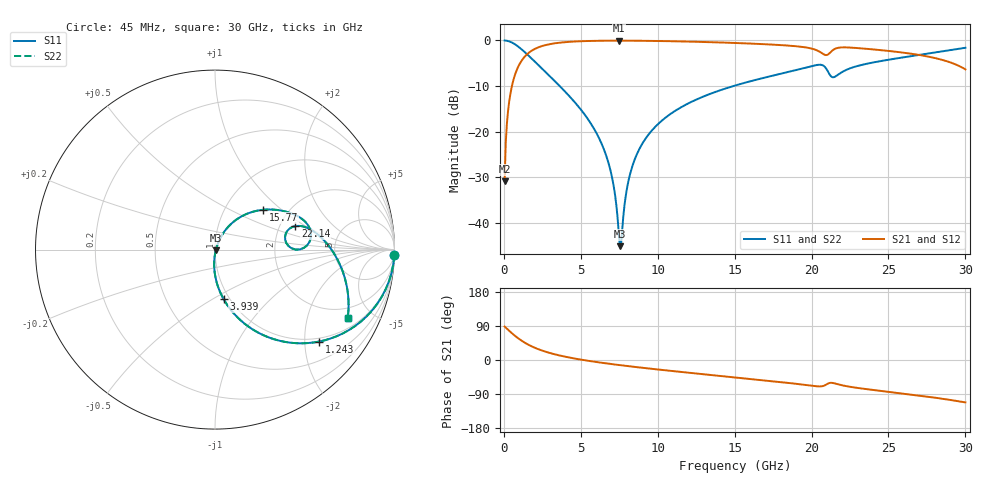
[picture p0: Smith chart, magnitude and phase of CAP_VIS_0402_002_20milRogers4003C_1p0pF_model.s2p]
! S-parameter model data by Modelithics Inc.  support@modelithics.com  813-866-6335  Tampa FL USA
! S-Parameter data specifications:
! Substrate: 20-mil Rogers 4003C, substrate thickness, H=0.508mm, Dielectric constant, Er=3.75
! PCB Mounting Pad Footprint: Pad width, PadW=0.50mm , Pad length, PadL=0.50mm , Pad gap, PadG (edge-to-edge)=0.40mm , Reference planes=1.4mm apart
! Created Wed Nov 18 12:37:36 2015
# hz S ma R 50
! 2 Port Network Data from SP1.SP block
! freq  magS11  angS11  magS21  angS21  magS12  angS12  magS22  angS22
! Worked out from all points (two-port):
!   401 points, 45 MHz to 30 GHz, reference 50 ohm
!   highest |S21| = -0.05 dB at 7.459 GHz (marker M1); lowest = -30.8 dB at 45 MHz (marker M2)
!   |S21| within 3 dB of the highest: 1.498 GHz to 20.8 GHz (19.3 GHz wide, 173 % of centre); 21.08 GHz to 26.75 GHz (5.668 GHz wide, 23.7 % of centre)
!   lowest |S11| = -45.1 dB at 7.534 GHz (marker M3), VSWR 1.01, Z = 50.5 - j0.322 ohm
!   |S11| at or under -10 dB: 3.629 GHz to 14.91 GHz (11.28 GHz wide, 122 % of centre)
!   |S22| runs from -45.1 to 0.0 dB; largest |S21 - S12| = 0
!   S11 on the Smith chart (normalised r, x): 45 MHz: 1, -66; 1.243 GHz: 0.91, -2.34; 3.939 GHz: 0.94, -0.56; 15.77 GHz: 1.50, +0.76; 22.14 GHz: 2.42, +0.81; 30 GHz: 1.46, -3.58
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4.5e7  0.9996 -1.7  0.02872 88.3  0.02872 88.3  0.9996 -1.7
2.696625e8  0.9854 -10.3  0.1699 79.7  0.1699 79.7  0.9854 -10.3
4.194375e8  0.9657 -15.8  0.2594 74.2  0.2594 74.2  0.9657 -15.8
1.2432e9  0.7745 -41.4  0.6312 48.5  0.6312 48.5  0.7745 -41.4
2.4414e9  0.4983 -64.2  0.8644 25.5  0.8644 25.5  0.4983 -64.2
3.93915e9  0.2794 -80.2  0.9565 9.1  0.9565 9.1  0.2794 -80.2
5.062462e9  0.1699 -88.0  0.9812 0.6  0.9812 0.6  0.1699 -88.0
6.709988e9  0.05098 -93.7  0.9936 -9.2  0.9936 -9.2  0.05098 -93.7
7.159312e9  0.02405 -89.5  0.9944 -11.6  0.9944 -11.6  0.02405 -89.5
7.458862e9  0.008112 -63.5  0.9946 -13.1  0.9946 -13.1  0.008112 -63.5
7.53375e9  0.005586 -34.9  0.9946 -13.5  0.9946 -13.5  0.005586 -34.9
7.683525e9  0.008197 35.8  0.9945 -14.3  0.9945 -14.3  0.008197 35.8
8.057962e9  0.02702 62.4  0.994 -16.1  0.994 -16.1  0.02702 62.4
8.4324e9  0.0462 65.2  0.9931 -17.9  0.9931 -17.9  0.0462 65.2
1.007992e10  0.1241 61.8  0.9858 -25.4  0.9858 -25.4  0.1241 61.8
1.50225e10  0.3205 42.6  0.9385 -45.9  0.9385 -45.9  0.3205 42.6
1.577138e10  0.348 39.6  0.9282 -49.0  0.9282 -49.0  0.348 39.6
2.003996e10  0.5241 17.6  0.8115 -68.0  0.8115 -68.0  0.5241 17.6
2.10135e10  0.4729 0.1  0.6943 -63.4  0.6943 -63.4  0.4729 0.1
2.213681e10  0.4656 16.3  0.8398 -68.1  0.8398 -68.1  0.4656 16.3
2.505742e10  0.6171 4.0  0.766 -84.2  0.766 -84.2  0.6171 4.0
3e10  0.8311 -27.2  0.4821 -111.8  0.4821 -111.8  0.8311 -27.2
